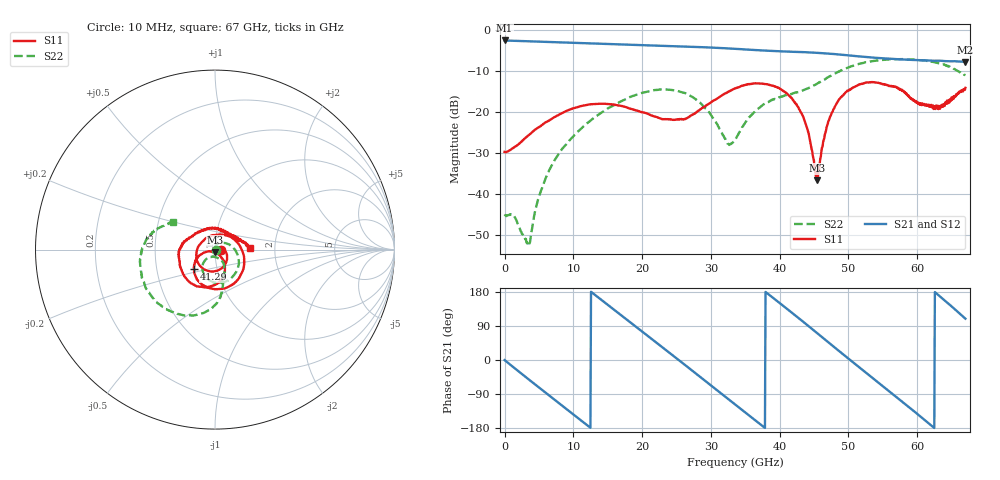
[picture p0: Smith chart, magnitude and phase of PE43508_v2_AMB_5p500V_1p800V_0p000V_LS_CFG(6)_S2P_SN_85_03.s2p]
!Keysight Technologies,N5227A,US51270237,A.10.43.00
!Date: Wednesday, August 22, 2018 17:07:08
!Correction: S11(Full 2 Port(1,3))
!S31(Full 2 Port(1,3))
!S13(Full 2 Port(1,3))
!S33(Full 2 Port(1,3))
!S2P File: Measurements: S11, S31, S13, S33:
# Hz S  dB  R 50
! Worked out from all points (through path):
!   801 points, 10 MHz to 67 GHz, reference 50 ohm
!   highest |S21| = -2.57 dB at 10 MHz (marker M1); lowest = -7.8 dB at 66.92 GHz (marker M2)
!   group delay of S21, straight-line fit = 40 ps
!   lowest |S11| = -36.8 dB at 45.48 GHz (marker M3), VSWR 1.03, Z = 49.9 - j1.45 ohm
!   |S11| at or under -10 dB: start of sweep to end of sweep
!   |S22| runs from -52.8 to -7.1 dB; largest |S21 - S12| = 0.005
!   S11 on the Smith chart (normalised r, x): 10 MHz: 1.07, -0.00; 41.29 GHz: 0.77, -0.17; 67 GHz: 1.49, +0.03
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1e7  -29.81 -0.9  -2.57 -0.2  -2.57 -0.2  -45.07 -8.9
3.526975e9  -25.74 -4.6  -2.78 -51.4  -2.78 -51.4  -52.37 50.1
6.37405e9  -22.23 -29.3  -2.92 -92.1  -2.92 -92.1  -34.74 83.9
1.123082e10  -18.56 -83.5  -3.19 -161.1  -3.19 -161.0  -23.99 35.7
1.40779e10  -18.04 -115.8  -3.36 158.7  -3.36 158.8  -20.23 9.4
1.734366e10  -18.70 -151.8  -3.56 112.6  -3.55 112.7  -17.13 -20.1
2.236791e10  -21.45 150.9  -3.85 41.8  -3.84 41.7  -14.61 -67.9
2.697348e10  -21.10 71.9  -4.10 -23.6  -4.10 -23.6  -16.07 -111.4
3.032298e10  -17.34 12.5  -4.34 -71.6  -4.33 -71.6  -21.57 -133.1
3.3505e10  -14.31 -36.0  -4.61 -117.3  -4.61 -117.2  -26.88 -76.9
3.735692e10  -13.14 -87.7  -5.00 -172.1  -4.99 -172.0  -18.60 -62.7
4.129259e10  -15.91 -137.2  -5.29 131.7  -5.29 131.8  -15.76 -75.3
4.346976e10  -21.45 -161.0  -5.43 100.1  -5.42 100.1  -14.69 -76.6
4.472582e10  -29.56 -164.0  -5.52 81.6  -5.51 81.7  -13.78 -77.6
4.547946e10  -36.76 -91.2  -5.60 70.5  -5.58 70.5  -13.07 -79.3
4.698674e10  -22.98 -51.0  -5.77 48.0  -5.76 48.0  -11.62 -83.3
4.874522e10  -16.80 -68.1  -6.01 22.1  -6.01 22.0  -10.06 -91.3
5.184351e10  -13.21 -106.2  -6.51 -23.3  -6.49 -23.4  -8.17 -109.9
5.586291e10  -13.72 -161.8  -7.01 -81.4  -7.01 -81.8  -7.19 -137.0
6.172454e10  -18.77 89.4  -7.48 -168.2  -7.51 -168.4  -7.62 -175.6
6.691626e10  -14.66 5.1  -7.80 110.5  -7.87 110.8  -10.99 147.4
6.7e10  -14.16 2.9  -7.80 109.1  -7.85 109.4  -11.06 146.1
